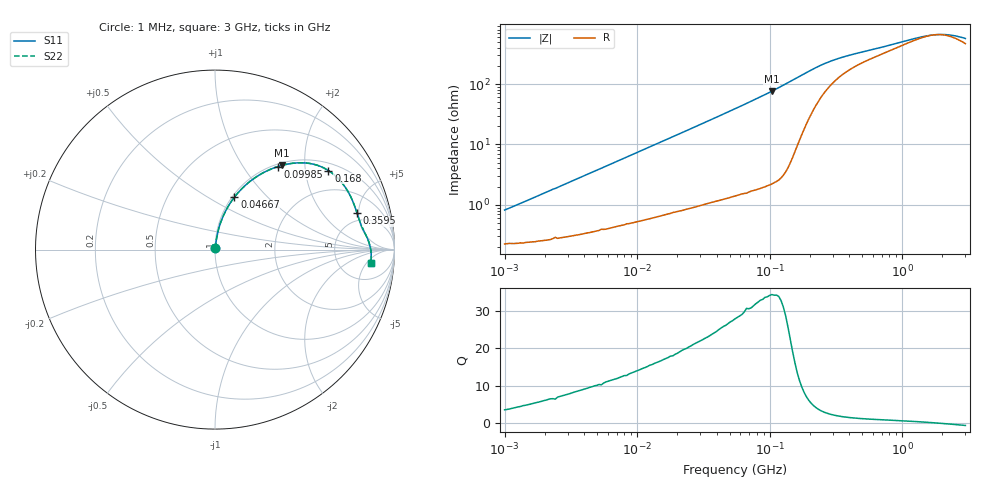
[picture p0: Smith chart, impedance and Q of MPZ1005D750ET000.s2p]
! S-Parameter Data Generated by TDK Corporation
! Copyright(C) 2025 TDK Corporation.
! All Rights Reserved.
! TDK P/N: MPZ1005D750ET000 (Chip Bead)
! Property: |Z|=75ohm at 100MHz
! Size(LxWxT): 1x0.5x0.5mm
! Model Type: s2p (Touchstone File Format Version 1.0)
! Frequency: DC=Yes Start=1MHz Stop=3000MHz 202points Log-sweep
! Model Generated on Feb. 6, 2025
! Terms and conditions regarding TDK Simulation Models:
! 1)This simulation model is being provided solely for informational
!  purposes. Please refer to the specifications of the products in
!  terms of detailed characteristics of such products.
! 2)In no event shall TDK Corporation of any of its subsidiaries be
!  liable for any loss or damage arising, directly or indirectly,
!  from any information contained in this simulation model, including,
!  but not limited to loss or damages arising from any inaccuracies,
!  omissions or errors in connection with such information.
! 3)Any and all copyrights on this simulation model are owned by
!  TDK Corporation.  Duplication or redistribution of this simulation
!  model without prior written permission from TDK Corporation
!  is prohibited.
! 4)This simulation model is subject to any modification or change
!  without any prior notice.
! 5)Neither TDK Corporation nor any of its subsidiaries shall make any
!  warranty, express or implied, including but not limited to the
!  correctness, implied warranties of merchantability and fitness for
!  a particular purpose with respect to this simulation models.
! 6)The use of this simulation model shall be deemed to have consented
!  to the terms and conditions hereof.
! Port Assignments:
!  1 ---@@@--- 2
! Applicable Conditions:
!  Temperature = 25 degC
!  DC Bias Current = 0 A
!  Small Signal Operation
# Hz S MA R 50
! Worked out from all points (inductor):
!   201 points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, 1 MHz to 3 GHz, reference 50 ohm
!   read as one part in series: L = 124 nH near 1.041 MHz
!   highest Q = 34.3 at 103.9 MHz (marker M1), where L = 117 nH
!   self-resonance near 1.777 GHz
!   S11 on the Smith chart (normalised r, x): 1 MHz: 1.00, +0.02; 46.67 MHz: 1.03, +0.66; 99.85 MHz: 1.04, +1.46; 168 MHz: 1.24, +2.67; 359.5 MHz: 3.94, +4.80; 3 GHz: 10, -6
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1000000  0.008141 73.6  0.9977 -0.4  0.9977 -0.4  0.008141 73.6
3900413  0.02955 81.9  0.9963 -1.7  0.9963 -1.7  0.02955 81.9
8017732  0.05894 82.1  0.9936 -3.4  0.9936 -3.4  0.05894 82.1
1.461624e7  0.1047 80.5  0.9882 -6.0  0.9882 -6.0  0.1047 80.5
2.886629e7  0.1999 75.8  0.9707 -11.5  0.9707 -11.5  0.1999 75.8
4.666789e7  0.3111 69.7  0.9386 -18.1  0.9386 -18.1  0.3111 69.7
5.477226e7  0.3585 67.0  0.9208 -21.0  0.9208 -21.0  0.3585 67.0
7.544761e7  0.4691 60.2  0.8684 -28.0  0.8684 -28.0  0.4691 60.2
9.984923e7  0.5806 52.8  0.7974 -35.5  0.7974 -35.5  0.5806 52.8
1.039275e8  0.5974 51.7  0.7848 -36.7  0.7848 -36.7  0.5974 51.7
1.321429e8  0.6972 43.8  0.6931 -44.2  0.6931 -44.2  0.6972 43.8
1.49005e8  0.7393 39.4  0.6359 -47.6  0.6359 -47.6  0.7393 39.4
1.680187e8  0.7702 34.9  0.5737 -50.1  0.5737 -50.1  0.7702 34.9
2.136344e8  0.8032 26.2  0.4511 -51.8  0.4511 -51.8  0.8032 26.2
2.609752e8  0.8125 20.4  0.3705 -49.9  0.3705 -49.9  0.8125 20.4
3.594878e8  0.8171 14.3  0.2905 -44.2  0.2905 -44.2  0.8171 14.3
4.951867e8  0.8231 10.5  0.2429 -38.2  0.2429 -38.2  0.8231 10.5
8.005644e8  0.8391 6.5  0.1912 -29.6  0.1912 -29.6  0.8391 6.5
1.294266e9  0.8587 2.7  0.1479 -15.9  0.1479 -15.9  0.8587 2.7
1.712864e9  0.8672 0.3  0.1329 -2.1  0.1329 -2.1  0.8672 0.3
2.266846e9  0.8713 -2.2  0.1338 14.8  0.1338 14.8  0.8713 -2.2
3e9  0.8704 -5.0  0.153 29.7  0.153 29.7  0.8704 -5.0
